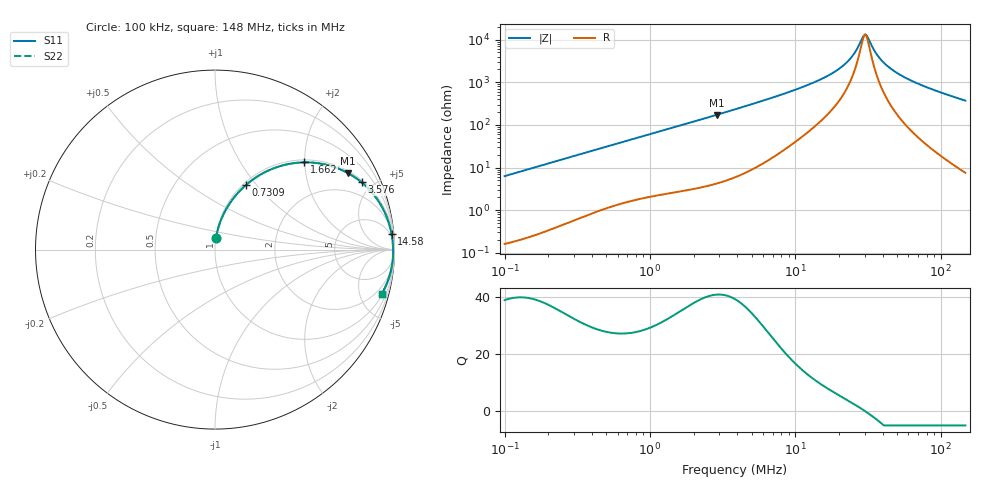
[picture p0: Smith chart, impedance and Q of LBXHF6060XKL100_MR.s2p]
! LBXHF6060XKL100_MR  S-PARAMETER MODEL  ( General Type )
! Model Generated by TAIYO YUDEN Corporation (http://www.ty-top.com)
! Version 1.0
! TAIYO YUDEN Control No. 220210
! Copyright(c) 2022 TAIYO YUDEN CO.,LTD. All Rights Reserved.
! Product Description (link to TY-COMPAS)
! https://ds.yuden.co.jp/TYCOMPAS/or/detail?pn=LBXHF6060XKL100MMR&u=M
! Products Name : Inductors
! Characteristics :
!  Inductance : 10 uH , SRF(min) : 20 MHz , DC Resistance(max) : 0.072 Ohm
!  Rated Current : Saturation :2200 mA , Temp Rise : 2700 mA
!  Case Size : 6.0 x 6.0 / 0.236 x 0.236 [mm/inch] , Thickness : 3 / 0.118 [mm/inch]
!  (Conditions: Temperature = 25 degC , DC Bias Current/Voltage = 0A / 0V)
! External Node Assignments :
!  1  o---GGG---o  2
! GND o---------o GND
! Frequency Range : 0.1MHz  -  147.97148MHz  [ 402 STEP ]
# MHz S RI R 50
! Freq[MHz].  S11 Real  S11 Imag  S21 Real  S21 Imag  S12 Real  S12 Imag  S22 Real  S22 Imag
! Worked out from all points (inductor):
!   401 points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, 100 kHz to 148 MHz, reference 50 ohm
!   read as one part in series: L = 10 uH near 103.7 kHz
!   highest Q = 40.8 at 2.873 MHz (marker M1), where L = 9.52 uH
!   self-resonance near 29.7 MHz
!   S11 on the Smith chart (normalised r, x): 100 kHz: 1.00, +0.13; 730.9 kHz: 1.03, +0.89; 1.662 MHz: 1.06, +1.98; 3.576 MHz: 1.11, +4.30; 14.58 MHz: 3, +22; 148 MHz: 1.15, -7.41
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0.1  0.00554 0.0625  0.9945 -0.0625  0.9945 -0.0625  0.00554 0.0625
0.339629  0.0484 0.1991  0.9516 -0.1991  0.9516 -0.1991  0.0484 0.1991
0.730926  0.1734 0.3608  0.8266 -0.3608  0.8266 -0.3608  0.1734 0.3608
1.153479  0.3292 0.4539  0.6708 -0.4539  0.6708 -0.4539  0.3292 0.4539
1.66157  0.4962 0.4861  0.5038 -0.4861  0.5038 -0.4861  0.4962 0.4861
2.872645  0.742 0.4254  0.258 -0.4254  0.258 -0.4254  0.742 0.4254
3.575915  0.8162 0.375  0.1838 -0.375  0.1838 -0.375  0.8162 0.375
3.917549  0.8419 0.3523  0.1581 -0.3523  0.1581 -0.3523  0.8419 0.3523
6.530207  0.9358 0.2275  0.0642 -0.2275  0.0642 -0.2275  0.9358 0.2275
13.06453  0.9806 0.1015  0.0194 -0.1015  0.0194 -0.1015  0.9806 0.1015
14.57627  0.9836 0.0862  0.0164 -0.0862  0.0164 -0.0862  0.9836 0.0862
18.81927  0.9885 0.0538  0.0115 -0.0538  0.0115 -0.0538  0.9885 0.0538
22.58693  0.9907 0.0326  0.00929 -0.0326  0.00929 -0.0326  0.9907 0.0326
25.20054  0.9916 0.0202  0.00837 -0.0202  0.00837 -0.0202  0.9916 0.0202
29.16174  0.9924 0.00402  0.00761 -0.00402  0.00761 -0.00402  0.9924 0.00402
30.24575  0.9925 -3.71e-05  0.0075 3.71e-05  0.0075 3.71e-05  0.9925 -3.71e-05
31.37005  0.9926 -0.0041  0.00743 0.0041  0.00743 0.0041  0.9926 -0.0041
36.96955  0.9925 -0.0226  0.00752 0.0226  0.00752 0.0226  0.9925 -0.0226
44.37094  0.9914 -0.0441  0.00856 0.0441  0.00856 0.0441  0.9914 -0.0441
54.23486  0.9889 -0.0694  0.0111 0.0694  0.0111 0.0694  0.9889 -0.0694
70.02204  0.9828 -0.1055  0.0172 0.1055  0.0172 0.1055  0.9828 -0.1055
147.9715  0.9277 -0.2491  0.0723 0.2491  0.0723 0.2491  0.9277 -0.2491
